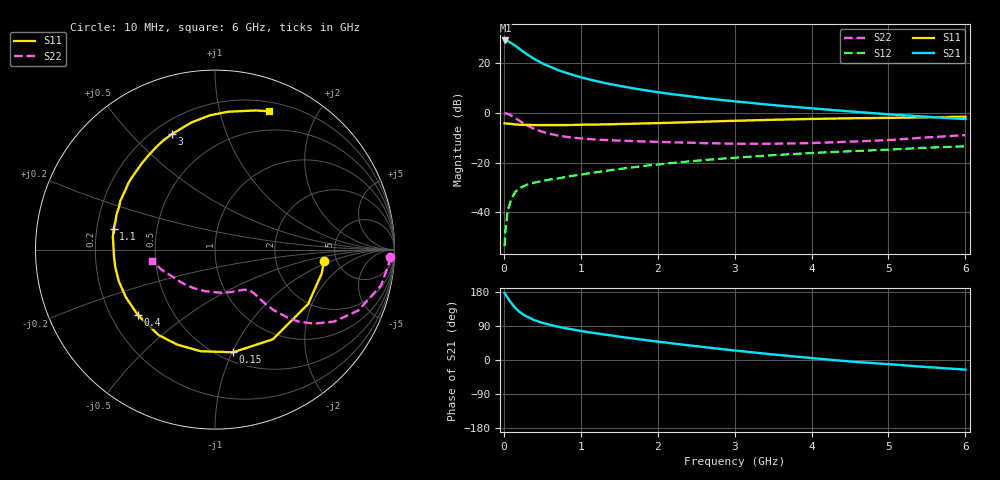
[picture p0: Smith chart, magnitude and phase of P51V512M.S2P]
! SIEMENS Small Signal Semiconductors
! BFP183
! Si NPN RF Bipolar Junction Transistor in SOT143
! VCE = 1.5 V  IC = 12 mA
! Common Emitter S-Parameters:  March  1996
# GHz  S  MA  R  50
!  f  S11  S21  S12  S22
! GHz  MAG  ANG  MAG  ANG  MAG  ANG  MAG  ANG
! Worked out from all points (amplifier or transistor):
!   36 points, 10 MHz to 6 GHz, reference 50 ohm
!   highest |S21| = 29.0 dB at 20 MHz (marker M1)
!   |S21| within 3 dB of that: start of sweep to 187 MHz
!   unconditionally stable (mu >= 1): 975.1 MHz to 5.643 GHz
!   at 250 MHz: K = 0.38, MSG = 27.1 dB, |S12| = -29.6 dB
!   at 1.4 GHz: K = 1.13, MAG = 15.0 dB, |S12| = -23.0 dB
!   at 6 GHz: K = 0.96, MSG = 5.5 dB, |S12| = -13.5 dB
!   S11 on the Smith chart (normalised r, x): 10 MHz: 3.95, -0.83; 150 MHz: 0.58, -1.01; 400 MHz: 0.31, -0.33; 1.1 GHz: 0.27, +0.09; 3 GHz: 0.27, +0.66; 6 GHz: 0.29, +1.42
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0.01  0.6102 -6.2  28 176.8  0.0021 83.8  0.9779 -2.4
0.02  0.6092 -12.6  28.07 173.7  0.0042 85.2  0.9704 -5.0
0.05  0.6009 -30.3  27.29 163.7  0.0107 78.9  0.9461 -12.3
0.1  0.5947 -57.2  24.67 149.4  0.0191 65.2  0.8676 -23.0
0.15  0.5807 -80.0  21.93 137.2  0.0258 58.3  0.776 -31.1
0.2  0.572 -98.0  19.19 127.8  0.0302 52.7  0.6904 -36.7
0.25  0.5696 -111.7  16.78 120.3  0.033 48.3  0.6173 -40.6
0.3  0.5706 -123.4  14.86 114.5  0.036 45.9  0.5558 -43.1
0.4  0.5635 -139.9  11.87 105.0  0.0396 43.4  0.4695 -45.9
0.5  0.5633 -152.0  9.756 98.2  0.0426 42.5  0.4141 -47.1
0.6  0.5642 -161.7  8.349 92.7  0.0457 42.5  0.3756 -47.6
0.7  0.5642 -169.7  7.18 88.0  0.048 42.8  0.3482 -47.9
0.9  0.5658 178.5  5.701 80.5  0.0546 44.0  0.3153 -48.7
1.1  0.5762 168.4  4.697 73.4  0.0607 45.0  0.2957 -50.0
1.5  0.5928 153.1  3.457 61.6  0.0741 46.0  0.2747 -54.6
1.8  0.6076 142.8  2.875 53.7  0.0843 45.4  0.2648 -59.6
2.2  0.6295 130.6  2.339 43.6  0.0983 43.8  0.2542 -67.6
3  0.6863 110.6  1.688 25.1  0.1248 38.8  0.2382 -88.2
3.5  0.7202 100.6  1.419 14.6  0.1404 35.1  0.238 -103.2
4.5  0.7712 84.7  1.058 -4.0  0.1682 27.0  0.2614 -134.8
5.5  0.8081 73.6  0.828 -18.6  0.1989 19.6  0.3188 -159.4
6  0.827 68.7  0.743 -25.4  0.2114 15.1  0.3542 -170.1
